(* Logix 5000 AddOnInstructionDefinition export AMCI_3202_AOP_Manual_Move_CCW; software revision 20.03 *)

ADD_ON_INSTRUCTION AMCI_3202_AOP_Manual_Move_CCW   (* revision 1.0, vendor AMCI, ExecuteEnableInFalse *)
VAR_INPUT
   axis_status_bits : INT; {required}
   channel_number : INT; {required}
   _0_normal_1_S_Curve_Acceleration : BOOL;
   _0_Triangular_1_Trapezoidal_S_Curve : BOOL;
   Programmed_speed : DINT; {required}
   Acceleration : DINT; {required}
   Deceleration : DINT; {required}
END_VAR
VAR_IN_OUT
   AMCI_3202_output_data : AM:1756_3202:O:0; {required}
END_VAR
VAR_OUTPUT
   EN : BOOL; {access Read Only, visible}
   Manual_Move_CCW_occurring : BOOL; {access Read Only, visible}
   ER : BOOL; {access Read Only, visible}
END_VAR
VAR
   command_data_block : DINT[8]; {access None}
END_VAR

ROUTINE EnableInFalse   (* ladder *)
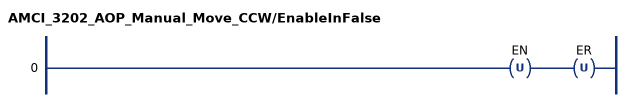
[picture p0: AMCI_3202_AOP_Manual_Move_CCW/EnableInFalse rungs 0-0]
   0: OTU(EN)OTU(ER);
END_ROUTINE

ROUTINE Logic   (* ladder *)
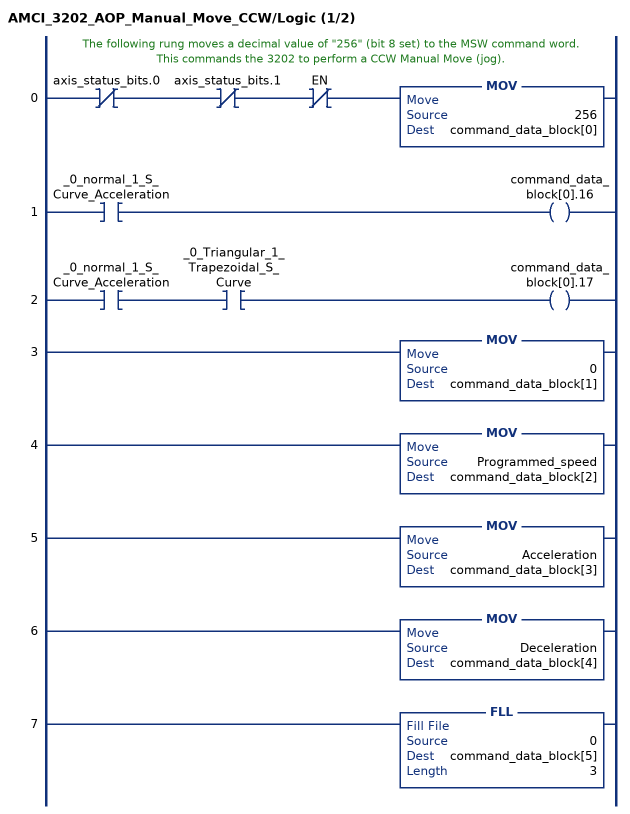
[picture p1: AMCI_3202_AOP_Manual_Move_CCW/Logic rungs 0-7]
   // The following rung moves a decimal value of "256" (bit 8 set) to the MSW command word.  This commands the 3202 to perform a CCW Manual Move (jog).
   0: XIO(axis_status_bits.0)XIO(axis_status_bits.1)XIO(EN)MOV(256,command_data_block[0]);
   1: XIC(_0_normal_1_S_Curve_Acceleration)OTE(command_data_block[0].16);
   2: XIC(_0_normal_1_S_Curve_Acceleration)XIC(_0_Triangular_1_Trapezoidal_S_Curve)OTE(command_data_block[0].17);
   3: MOV(0,command_data_block[1]);
   4: MOV(Programmed_speed,command_data_block[2]);
   5: MOV(Acceleration,command_data_block[3]);
   6: MOV(Deceleration,command_data_block[4]);
   7: FLL(0,command_data_block[5],3);
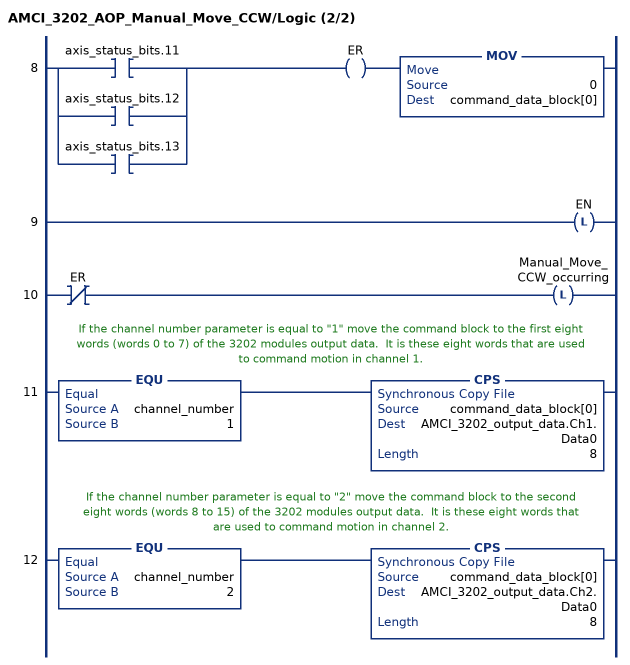
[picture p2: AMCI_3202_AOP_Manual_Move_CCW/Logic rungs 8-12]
   8: [XIC(axis_status_bits.11) ,XIC(axis_status_bits.12) ,XIC(axis_status_bits.13) ]OTE(ER)MOV(0,command_data_block[0]);
   9: OTL(EN);
   10: XIO(ER)OTL(Manual_Move_CCW_occurring);
   // If the channel number parameter is equal to "1" move the command block to the first eight words (words 0 to 7) of the 3202 modules output data.  It is these eight words that are used to command motion in channel 1.
   11: EQU(channel_number,1)CPS(command_data_block[0],AMCI_3202_output_data.Ch1.Data0,8);
   // If the channel number parameter is equal to "2" move the command block to the second eight words (words 8 to 15) of the 3202 modules output data.  It is these eight words that are used to command motion in channel 2.
   12: EQU(channel_number,2)CPS(command_data_block[0],AMCI_3202_output_data.Ch2.Data0,8);
END_ROUTINE
END_ADD_ON_INSTRUCTION
